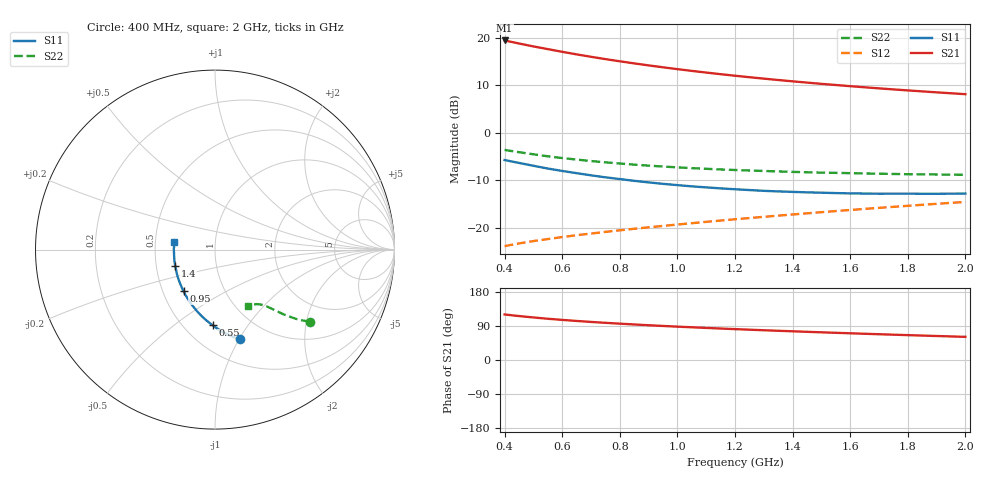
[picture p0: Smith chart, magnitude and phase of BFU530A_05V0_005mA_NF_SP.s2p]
! Filename:  P:\Prog\Test\Noise\ATS_data\Testdata_Net\06 Compressed Noise after Statistics\BFU530A_APG2013_33_A05_05p0V_005mA_NF_CM01_D.sf
! Date/Time: Tue 16/Apr/2013 15:10:56
! BFU530A_APG2013_33_A05_05p0V_1to25mA_NF_CM01_Bias4_R.sf
! Noise Parameter Data File
! BFU530A_APG2013_33_A05_05p0V_1to25mA_NF_CM01
! Date/time: Fri Apr 12 15:27:54 2013
! VAR V_out= 5.001000
! VAR I_out= 5.000000
! VAR V_in= 0.819900
! VAR I_in= 0.052900
! Device data file deembeded for feedlines and parallel
! Original file: \06 Compressed Noise after Statistics\BFU530A_APG2013_33_A05_05p0V_005mA_NF_CM01_R.sf
! Feed-files: PR017V01_150413_Feed1.s2p, PR017V01_150413_Feed2.s2p
! Parallel-file: PR017V01_150413_Par.s2p
# MHz S MA R 50
!  Freq-MHz  S11-mag  S11-arg  S21-mag  S21-arg  S12-mag  S12-arg  S22-mag  S22-arg
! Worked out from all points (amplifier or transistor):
!   37 points, 400 MHz to 2 GHz, reference 50 ohm
!   highest |S21| = 19.5 dB at 400 MHz (marker M1)
!   |S21| within 3 dB of that: start of sweep to 656.8 MHz
!   unconditionally stable (mu >= 1): 1.61 GHz to end of sweep
!   at 500 MHz: K = 0.61, MSG = 20.5 dB, |S12| = -22.8 dB
!   at 1.1 GHz: K = 0.92, MSG = 15.7 dB, |S12| = -18.7 dB
!   at 2 GHz: K = 1.01, MAG = 10.6 dB, |S12| = -14.5 dB
!   lowest NFmin = 0.60 dB at 420 MHz
!   S11 on the Smith chart (normalised r, x): 400 MHz: 0.74, -1.01; 550 MHz: 0.68, -0.70; 950 MHz: 0.64, -0.32; 1.4 GHz: 0.63, -0.12; 2 GHz: 0.63, +0.05
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400  0.5187 -74.4  9.413 120.2  0.06421 60.1  0.6624 -37.2
420  0.5039 -76.9  9.136 118.4  0.06601 59.6  0.6474 -38.0
440  0.4896 -79.5  8.877 116.8  0.06772 59.3  0.6338 -38.7
480  0.4639 -84.1  8.375 113.7  0.07104 58.8  0.6077 -39.9
500  0.4512 -86.3  8.146 112.3  0.07266 58.5  0.5961 -40.4
550  0.4217 -91.9  7.631 108.8  0.07629 58.1  0.5671 -41.6
600  0.3978 -96.8  7.146 105.8  0.08006 58.0  0.5441 -42.5
650  0.377 -101.6  6.717 103.1  0.08376 57.9  0.5242 -43.4
700  0.3578 -106.2  6.336 100.5  0.08722 58.0  0.506 -44.1
750  0.3408 -110.6  5.987 98.1  0.0908 58.1  0.4899 -44.7
800  0.3268 -114.9  5.679 95.9  0.09433 58.2  0.4762 -45.3
850  0.3129 -119.0  5.398 93.7  0.09785 58.4  0.4634 -45.8
900  0.3015 -123.2  5.142 91.7  0.1014 58.6  0.4526 -46.4
950  0.2909 -127.0  4.909 89.8  0.1049 58.9  0.4427 -46.9
1050  0.2738 -134.4  4.5 86.3  0.1121 59.4  0.4258 -47.8
1200  0.2554 -145.1  4.003 81.5  0.1232 60.0  0.407 -49.3
1300  0.2456 -151.5  3.731 78.5  0.1308 60.3  0.3976 -50.3
1400  0.2396 -158.0  3.494 75.7  0.1385 60.6  0.389 -51.5
1500  0.2348 -164.2  3.287 73.0  0.1463 60.8  0.382 -52.7
1650  0.2301 -172.6  3.025 69.2  0.1585 61.0  0.3745 -54.6
1750  0.2293 -178.2  2.873 66.8  0.1666 61.0  0.3697 -56.0
2000  0.23 169.7  2.559 61.1  0.1878 60.8  0.3624 -59.8
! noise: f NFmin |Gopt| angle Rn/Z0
400  0.6467  0.1869  21.23  0.1195
460  0.6372  0.1444  29.79  0.1072
600  0.7242  0.1877  30.15  0.1258
800  0.6848  0.1542  64.9  0.0974
1000  0.7147  0.1662  79.89  0.0935
1200  0.7568  0.1704  93.6  0.093
1400  0.7818  0.1723  115.7  0.0889
1600  0.8203  0.1817  135.1  0.0744
1800  0.7601  0.1852  153.2  0.0753
2000  0.8134  0.2141  171.5  0.065
